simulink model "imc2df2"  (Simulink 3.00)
settings: Solver=ode45  SolverMode=SingleTasking  StartTime=0.0  StopTime=10  FixedStep=st_size  MaxStep=st_size  RelTol=1e-5  AbsTol=1e-6
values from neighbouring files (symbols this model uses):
  d_through_p = get(MAIN_MENU(19),'Value')    [cback.m]    (also in imcmenu.m = 0)
  Disturb = Setpoint    [mimo_MSF1DF_sim.m]    (also in mimo_MSF2DF_sim.m)
  qdden = 1    [FindTwo.m]
  qdnum = 1    [FindTwo.m]
  Satlb = temp1    [cback.m]    (also in imcmenu.m = str2num(satlbs))
  Satub = temp1    [cback.m]    (also in imcmenu.m = str2num(satubs))
  Setpoint = zeros(1,n)    [mimo_MSF1DF_sim.m]    (also in mimo_MSF2DF_sim.m)
undefined symbols (not defined in the file or in its folder): denCs, denCs2, denPd, mdeadx, numCs, numCs2, numPd, pdeadx, XdenMs, XdenPs, XnumMs, XnumPs

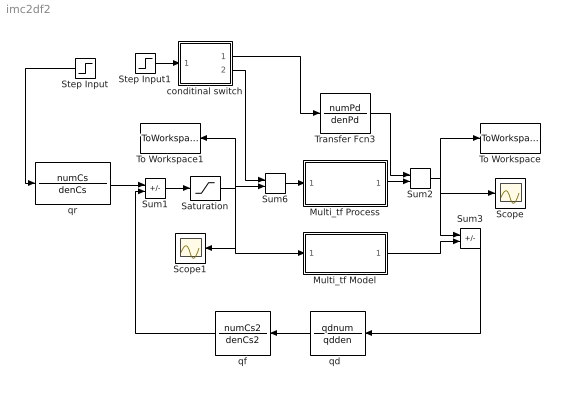
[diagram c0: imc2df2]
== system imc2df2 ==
  Multi_tf Model : Subsystem
  Multi_tf Process : Subsystem
  Saturation : Saturate  UpperLimit=Satub  LowerLimit=Satlb
  Scope : Scope
  Scope1 : Scope
  Step Input : Step  Orientation=left  Time=0  Before=0  After=Setpoint  SampleTime=0
  Step Input1 : Step  Time=0  Before=0  After=Disturb  SampleTime=0
  Sum1 : Sum  Inputs=+-  SaturateOnIntegerOverflow=on
  Sum2 : Sum  Inputs=++  SaturateOnIntegerOverflow=on
  Sum3 : Sum  Inputs=+-  SaturateOnIntegerOverflow=on
  Sum6 : Sum  Inputs=++  SaturateOnIntegerOverflow=on
  To Workspace : ToWorkspace  VariableName=simout  SampleTime=-1  SaveFormat=Matrix
  To Workspace1 : ToWorkspace  VariableName=effort  SampleTime=-1  SaveFormat=Matrix
  Transfer Fcn3 : TransferFcn  Numerator=numPd  Denominator=denPd
  conditinal switch : Subsystem  Description=pass input signal through out1 if condition is true.
  "qd  " : TransferFcn  Orientation=left  Numerator=qdnum  Denominator=qdden
  qf : TransferFcn  Orientation=left  Numerator=numCs2  Denominator=denCs2
  qr : TransferFcn  Numerator=numCs  Denominator=denCs
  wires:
  Step Input/1 -> qr/1
  qr/1 -> Sum1/1
  Sum3/1 -> "qd  "/1
  "qd  "/1 -> qf/1
  qf/1 -> Sum1/2
  Sum1/1 -> Saturation/1
  Multi_tf Model/1(Out1) -> Sum3/2
  Saturation/1 -> Sum6/2, Multi_tf Model/1(In1), Scope1/1, To Workspace1/1
  conditinal switch/2(Out1) -> Sum6/1
  conditinal switch/1(Out2) -> Transfer Fcn3/1
  Step Input1/1 -> conditinal switch/1(In)
  Sum6/1 -> Multi_tf Process/1(In1)
  Multi_tf Process/1(Out1) -> Sum2/2
  Transfer Fcn3/1 -> Sum2/1
  Sum2/1 -> Sum3/1, To Workspace/1, Scope/1

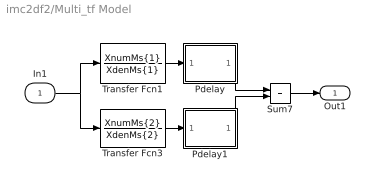
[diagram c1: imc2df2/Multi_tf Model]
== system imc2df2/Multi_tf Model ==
  In1 : Inport  Port=1  PortWidth=-1  SampleTime=-1  DataType=auto
  Pdelay : Subsystem
  Pdelay1 : Subsystem
  Sum7 : Sum  Inputs=++  SaturateOnIntegerOverflow=on
  Transfer Fcn1 : TransferFcn  Numerator=XnumMs{1}  Denominator=XdenMs{1}
  Transfer Fcn3 : TransferFcn  Numerator=XnumMs{2}  Denominator=XdenMs{2}
  Out1 : Outport  Port=1  InitialOutput=0
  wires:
  Transfer Fcn1/1 -> Pdelay/1(In1)
  Transfer Fcn3/1 -> Pdelay1/1(In1)
  In1/1 -> Transfer Fcn1/1, Transfer Fcn3/1
  Sum7/1 -> Out1/1
  Pdelay/1(Out1) -> Sum7/1
  Pdelay1/1(Out1) -> Sum7/2

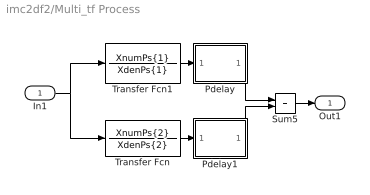
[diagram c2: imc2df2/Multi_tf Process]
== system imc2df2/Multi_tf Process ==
  In1 : Inport  Port=1  PortWidth=-1  SampleTime=-1  DataType=auto
  Pdelay : Subsystem
  Pdelay1 : Subsystem
  Sum5 : Sum  Inputs=++  SaturateOnIntegerOverflow=on
  Transfer Fcn : TransferFcn  Numerator=XnumPs{2}  Denominator=XdenPs{2}
  Transfer Fcn1 : TransferFcn  Numerator=XnumPs{1}  Denominator=XdenPs{1}
  Out1 : Outport  Port=1  InitialOutput=0
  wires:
  Transfer Fcn1/1 -> Pdelay/1(In1)
  Transfer Fcn/1 -> Pdelay1/1(In1)
  In1/1 -> Transfer Fcn1/1, Transfer Fcn/1
  Sum5/1 -> Out1/1
  Pdelay/1(Out1) -> Sum5/1
  Pdelay1/1(Out1) -> Sum5/2

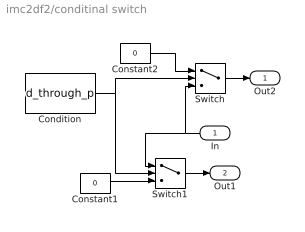
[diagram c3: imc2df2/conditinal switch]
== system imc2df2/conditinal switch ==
  In : Inport  Orientation=left  Port=1  PortWidth=-1  SampleTime=-1  DataType=auto
  Condition : Constant  Value=d_through_p
  Constant1 : Constant  Value=0
  Constant2 : Constant  Value=0
  Switch : Switch  Threshold=1
  Switch1 : Switch  Threshold=1
  Out2 : Outport  Port=1  InitialOutput=0
  Out1 : Outport  Port=2  InitialOutput=0
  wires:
  In/1 -> Switch/3, Switch1/1
  Condition/1 -> Switch1/2, Switch/2
  Constant1/1 -> Switch1/3
  Constant2/1 -> Switch/1
  Switch/1 -> Out2/1
  Switch1/1 -> Out1/1

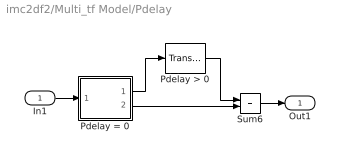
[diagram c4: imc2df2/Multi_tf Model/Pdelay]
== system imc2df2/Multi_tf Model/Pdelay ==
  In1 : Inport  Port=1  PortWidth=-1  SampleTime=-1  DataType=auto
  Pdelay > 0 : TransportDelay  DelayTime=mdeadx(1)  InitialInput=0  BufferSize=1024
  Pdelay = 0 : Subsystem  Description=pass input signal through out1 if condition is true.
  Sum6 : Sum  Inputs=++  SaturateOnIntegerOverflow=on
  Out1 : Outport  Port=1
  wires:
  Pdelay = 0/1(Out2) -> Pdelay > 0/1
  Pdelay > 0/1 -> Sum6/1
  Pdelay = 0/2(Out1) -> Sum6/2
  In1/1 -> Pdelay = 0/1(In)
  Sum6/1 -> Out1/1

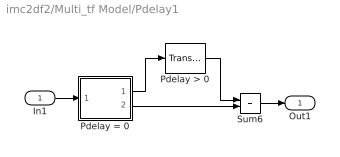
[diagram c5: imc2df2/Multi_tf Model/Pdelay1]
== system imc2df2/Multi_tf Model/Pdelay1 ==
  In1 : Inport  Port=1  PortWidth=-1  SampleTime=-1  DataType=auto
  Pdelay > 0 : TransportDelay  DelayTime=mdeadx(2)  InitialInput=0  BufferSize=1024
  Pdelay = 0 : Subsystem  Description=pass input signal through out1 if condition is true.
  Sum6 : Sum  Inputs=++  SaturateOnIntegerOverflow=on
  Out1 : Outport  Port=1
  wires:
  Pdelay = 0/1(Out2) -> Pdelay > 0/1
  Pdelay > 0/1 -> Sum6/1
  Pdelay = 0/2(Out1) -> Sum6/2
  In1/1 -> Pdelay = 0/1(In)
  Sum6/1 -> Out1/1

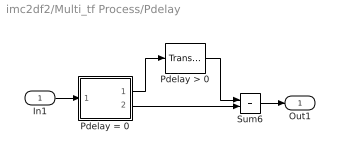
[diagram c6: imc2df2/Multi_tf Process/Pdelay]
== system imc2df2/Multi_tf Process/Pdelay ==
  In1 : Inport  Port=1  PortWidth=-1  SampleTime=-1  DataType=auto
  Pdelay > 0 : TransportDelay  DelayTime=pdeadx(1)  InitialInput=0  BufferSize=1024
  Pdelay = 0 : Subsystem  Description=pass input signal through out1 if condition is true.
  Sum6 : Sum  Inputs=++  SaturateOnIntegerOverflow=on
  Out1 : Outport  Port=1
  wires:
  Pdelay = 0/1(Out2) -> Pdelay > 0/1
  Pdelay > 0/1 -> Sum6/1
  Pdelay = 0/2(Out1) -> Sum6/2
  In1/1 -> Pdelay = 0/1(In)
  Sum6/1 -> Out1/1

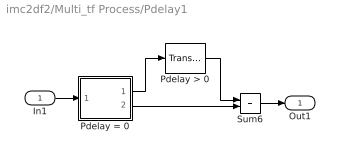
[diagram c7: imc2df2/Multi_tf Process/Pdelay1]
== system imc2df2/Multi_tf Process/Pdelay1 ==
  In1 : Inport  Port=1  PortWidth=-1  SampleTime=-1  DataType=auto
  Pdelay > 0 : TransportDelay  DelayTime=pdeadx(2)  InitialInput=0  BufferSize=1024
  Pdelay = 0 : Subsystem  Description=pass input signal through out1 if condition is true.
  Sum6 : Sum  Inputs=++  SaturateOnIntegerOverflow=on
  Out1 : Outport  Port=1
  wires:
  Pdelay = 0/1(Out2) -> Pdelay > 0/1
  Pdelay > 0/1 -> Sum6/1
  Pdelay = 0/2(Out1) -> Sum6/2
  In1/1 -> Pdelay = 0/1(In)
  Sum6/1 -> Out1/1

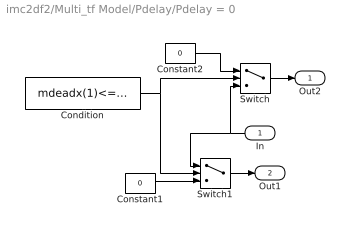
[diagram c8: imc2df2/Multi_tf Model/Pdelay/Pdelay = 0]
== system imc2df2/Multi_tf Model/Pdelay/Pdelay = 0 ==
  In : Inport  Orientation=left  Port=1  PortWidth=-1  SampleTime=-1  DataType=auto
  Condition : Constant  Value=mdeadx(1)<=3*eps
  Constant1 : Constant  Value=0
  Constant2 : Constant  Value=0
  Switch : Switch  Threshold=1
  Switch1 : Switch  Threshold=1
  Out2 : Outport  Port=1  InitialOutput=0
  Out1 : Outport  Port=2  InitialOutput=0
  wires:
  In/1 -> Switch/3, Switch1/1
  Condition/1 -> Switch1/2, Switch/2
  Constant1/1 -> Switch1/3
  Constant2/1 -> Switch/1
  Switch/1 -> Out2/1
  Switch1/1 -> Out1/1

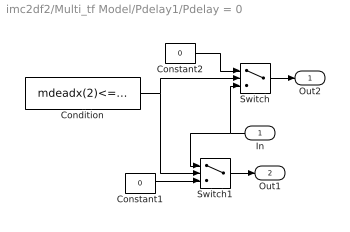
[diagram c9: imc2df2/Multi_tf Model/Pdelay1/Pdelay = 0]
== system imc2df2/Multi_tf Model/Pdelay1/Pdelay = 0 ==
  In : Inport  Orientation=left  Port=1  PortWidth=-1  SampleTime=-1  DataType=auto
  Condition : Constant  Value=mdeadx(2)<=3*eps
  Constant1 : Constant  Value=0
  Constant2 : Constant  Value=0
  Switch : Switch  Threshold=1
  Switch1 : Switch  Threshold=1
  Out2 : Outport  Port=1  InitialOutput=0
  Out1 : Outport  Port=2  InitialOutput=0
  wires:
  In/1 -> Switch/3, Switch1/1
  Condition/1 -> Switch1/2, Switch/2
  Constant1/1 -> Switch1/3
  Constant2/1 -> Switch/1
  Switch/1 -> Out2/1
  Switch1/1 -> Out1/1

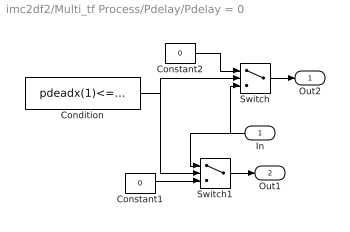
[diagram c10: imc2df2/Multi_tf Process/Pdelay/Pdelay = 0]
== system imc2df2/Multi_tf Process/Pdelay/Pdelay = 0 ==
  In : Inport  Orientation=left  Port=1  PortWidth=-1  SampleTime=-1  DataType=auto
  Condition : Constant  Value=pdeadx(1)<=3*eps
  Constant1 : Constant  Value=0
  Constant2 : Constant  Value=0
  Switch : Switch  Threshold=1
  Switch1 : Switch  Threshold=1
  Out2 : Outport  Port=1  InitialOutput=0
  Out1 : Outport  Port=2  InitialOutput=0
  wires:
  In/1 -> Switch/3, Switch1/1
  Condition/1 -> Switch1/2, Switch/2
  Constant1/1 -> Switch1/3
  Constant2/1 -> Switch/1
  Switch/1 -> Out2/1
  Switch1/1 -> Out1/1

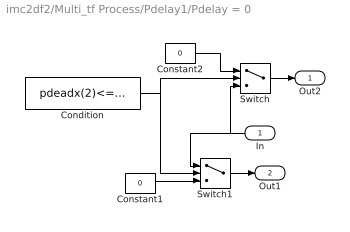
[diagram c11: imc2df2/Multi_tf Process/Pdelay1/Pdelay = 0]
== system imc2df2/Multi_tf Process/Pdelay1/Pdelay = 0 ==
  In : Inport  Orientation=left  Port=1  PortWidth=-1  SampleTime=-1  DataType=auto
  Condition : Constant  Value=pdeadx(2)<=3*eps
  Constant1 : Constant  Value=0
  Constant2 : Constant  Value=0
  Switch : Switch  Threshold=1
  Switch1 : Switch  Threshold=1
  Out2 : Outport  Port=1  InitialOutput=0
  Out1 : Outport  Port=2  InitialOutput=0
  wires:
  In/1 -> Switch/3, Switch1/1
  Condition/1 -> Switch1/2, Switch/2
  Constant1/1 -> Switch1/3
  Constant2/1 -> Switch/1
  Switch/1 -> Out2/1
  Switch1/1 -> Out1/1
